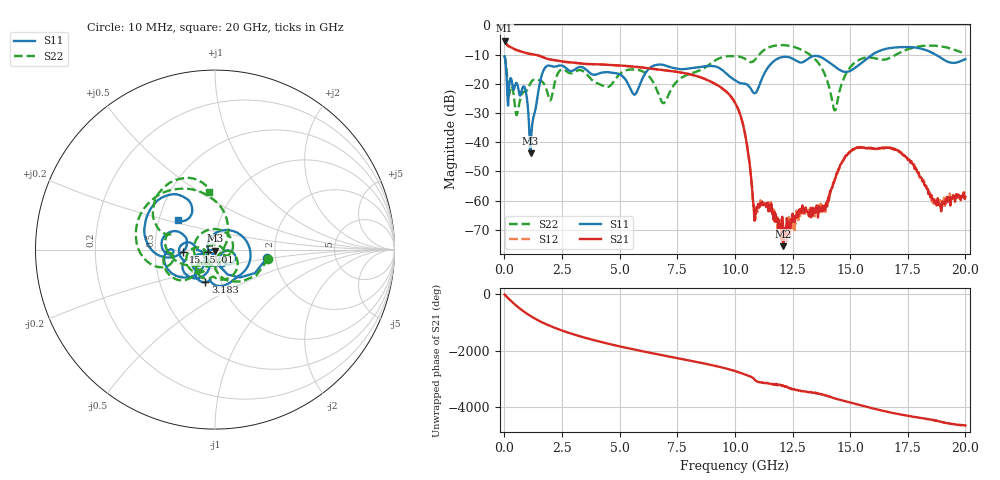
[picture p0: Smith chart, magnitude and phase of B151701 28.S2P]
!  2-Port S-parameters saved by WinCal
! VAR MeasName=S-Parameters (CALIBRATED_DATA) read from VNA (N5244A)
! VAR MeasDate=2015-12-24 19:11:22
! VAR NAME=B151701 28
! VAR FILENAME=B151701 28.S2P
! VAR DATE=2015-12-24 19:11:22
! VAR PHYS_PORTS=1,3
# Hz S DB R 50
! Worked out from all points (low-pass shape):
!   801 points, 10 MHz to 20 GHz, reference 50 ohm
!   highest |S21| = -5.20 dB at 10 MHz (marker M1); lowest = -75.6 dB at 12.1 GHz (marker M2)
!   |S21| within 3 dB of the highest: start of sweep to 446.6 MHz
!   lowest |S11| = -43.8 dB at 1.134 GHz (marker M3), VSWR 1.01, Z = 49.9 - j0.634 ohm
!   |S11| at or under -10 dB: start of sweep to 15.97 GHz; 18.7 GHz to end of sweep
!   |S22| runs from -30.8 to -6.8 dB; largest |S21 - S12| = 0.0014
!   S11 on the Smith chart (normalised r, x): 10 MHz: 1.80, -0.19; 1.01 GHz: 0.92, -0.03; 3.183 GHz: 0.84, -0.32; 15.15 GHz: 0.70, -0.02; 20 GHz: 0.63, +0.22
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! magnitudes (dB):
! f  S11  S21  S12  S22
! 10 MHz  -10.7  -5.2  -5.2  -10.4
! 184.9 MHz  -23.6  -7.1  -7.1  -23.6
! 534.7 MHz  -19.7  -8.5  -8.5  -30.8
! 1.01 GHz  -27.2  -9.6  -9.6  -21.9
! 1.134 GHz  -43.8  -9.8  -9.8  -19.8
! 1.759 GHz  -14.6  -11.2  -11.2  -20.6
! 3.183 GHz  -14.5  -12.9  -12.9  -15.4
! 3.358 GHz  -14.3  -13.1  -13.1  -15.5
! 4.458 GHz  -16.0  -13.5  -13.5  -21.1
! 5.632 GHz  -23.7  -14.1  -14.1  -15.1
! 6.682 GHz  -13.4  -15.1  -15.1  -23.4
! 10.01 GHz  -18.8  -26.5  -26.5  -10.6
! 10.45 GHz  -20.0  -37.7  -37.8  -11.5
! 10.88 GHz  -23.2  -64.0  -66.5  -11.7
! 11.5 GHz  -13.7  -61.5  -61.2  -7.4
! 12.1 GHz  -10.8  -75.6  -69.8  -6.8
! 13.35 GHz  -10.7  -65.3  -62.8  -10.7
! 14.33 GHz  -14.1  -53.0  -53.0  -29.1
! 15.15 GHz  -14.9  -42.3  -42.6  -13.1
! 16.68 GHz  -7.8  -41.9  -41.9  -11.3
! 18.85 GHz  -10.7  -61.3  -60.0  -7.1
! 20 GHz  -11.6  -58.7  -58.3  -9.8
